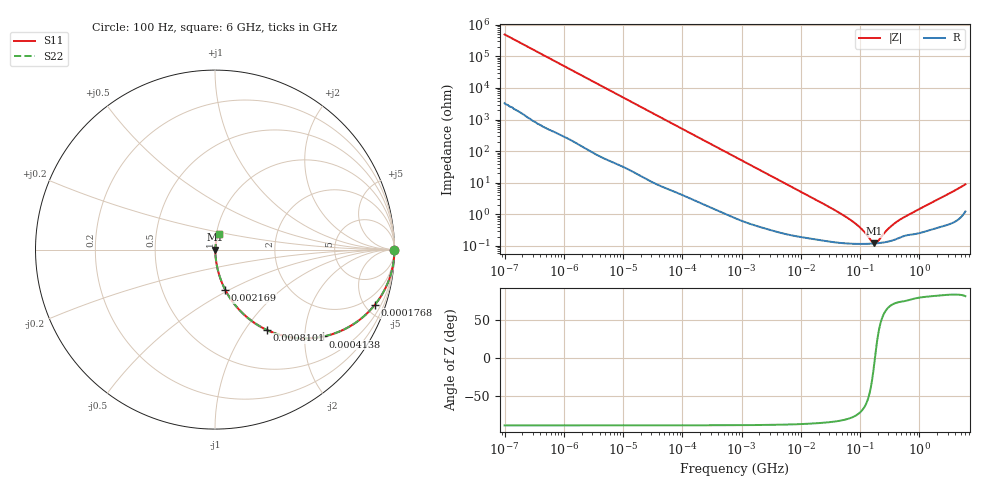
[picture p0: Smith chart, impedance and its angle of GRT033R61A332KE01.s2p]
!Murata Part Number: GRT033R61A332KE01
!These Parameters are Measured in Series Mode Connection
!Data Generated on Jun 19, 2026
!  o--ll--o
!Port1  Port2
!  o------o
!Operation Temp=25[degC], DC Bias Voltage=0[V]
!Freq. Start=100[Hz] Stop=6[GHz] 401[Steps]
# Hz S RI R 50
!Freq.(Hz) S11(Real) S11(Imag) S21(Real) S21(Imag) S12(Real) S12(Imag) S22(Real) S22(Imag)
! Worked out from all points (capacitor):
!   401 points, 100 Hz to 6 GHz, reference 50 ohm
!   read as one part in series: C = 3.21 nF near 109 Hz
!   lowest |Z| = 121 mohm at 174.6 MHz (marker M1)
!   series resonance near 178.5 MHz, so ESL is about 250 pH
!   S11 on the Smith chart (normalised r, x): 100 Hz: open; 176.8 kHz: 1.05, -5.76; 413.8 kHz: 1.03, -2.47; 810.1 kHz: 1.01, -1.27; 2.169 MHz: 1.01, -0.48; 6 GHz: 1.02, +0.18
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100  1 -0.000202  1.4e-06 0.000202  1.4e-06 0.000202  1 -0.000202
2008  1 -0.00402  3.91e-05 0.00402  3.91e-05 0.00402  1 -0.00402
40335  0.9932 -0.0792  0.00684 0.0792  0.00684 0.0792  0.9932 -0.0792
86348  0.9706 -0.165  0.0294 0.165  0.0294 0.165  0.9706 -0.165
176758  0.8903 -0.3081  0.1097 0.3081  0.1097 0.3081  0.8903 -0.3081
264476  0.786 -0.4054  0.214 0.4054  0.214 0.4054  0.786 -0.4054
413847  0.6035 -0.484  0.3965 0.484  0.3965 0.484  0.6035 -0.484
774597  0.3074 -0.4557  0.6926 0.4557  0.6926 0.4557  0.3074 -0.4557
810067  0.2891 -0.4476  0.7109 0.4476  0.7109 0.4476  0.2891 -0.4476
1267578  0.145 -0.3456  0.855 0.3456  0.855 0.3456  0.145 -0.3456
2169299  0.057 -0.2238  0.943 0.2238  0.943 0.2238  0.057 -0.2238
5079039  0.0128 -0.1008  0.9872 0.1008  0.9872 0.1008  0.0128 -0.1008
1.555665e7  0.0028 -0.0334  0.9972 0.0334  0.9972 0.0334  0.0028 -0.0334
4.165952e7  0.00142 -0.0121  0.9986 0.0121  0.9986 0.0121  0.00142 -0.0121
7.455971e7  0.00121 -0.00592  0.9988 0.00592  0.9988 0.00592  0.00121 -0.00592
1.066761e8  0.00117 -0.00322  0.9988 0.00322  0.9988 0.00322  0.00117 -0.00322
1.526266e8  0.00118 -0.00094  0.9988 0.00094  0.9988 0.00094  0.00118 -0.00094
1.745687e8  0.0012 -0.00013  0.9988 0.00013  0.9988 0.00013  0.0012 -0.00013
1.996653e8  0.00123 0.000676  0.9988 -0.000676  0.9988 -0.000676  0.00123 0.000676
3.124326e8  0.00142 0.00351  0.9986 -0.00351  0.9986 -0.00351  0.00142 0.00351
5.346885e8  0.00208 0.00759  0.9979 -0.00759  0.9979 -0.00759  0.00208 0.00759
6e9  0.0198 0.0856  0.9802 -0.0856  0.9802 -0.0856  0.0198 0.0856
